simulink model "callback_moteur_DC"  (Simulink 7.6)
settings: Solver=ode15s  StartTime=0.0  StopTime=N  RelTol=1e-3
PostLoadFcn:
  | clc
  | clear all
  | close all
  | delete *.mat
InitFcn:
  | clc, clear all, close all
  | % Durée de simulation et temps de l'échelon
  | N=1;
  | % paramètres du moteur
  | R=3.9; % résistance d'induit
  | L=12e-6; % inductance d'induit
  | K=5e-4; % paramètre électromécanique
  | J=0.02; % inertie
  | Mr=0.02e-3; % frottements
StopFcn:
  | close all
  | load vit_pos_mot_DC.mat
  | plotyy(x(1,:),x(2,:), x(1,:),x(3,:))
  | grid
  | title('Position et Vitesse d''un moteur DC')
  | xlabel('temps')
libraries: fl_lib x10, nesl_utility x4

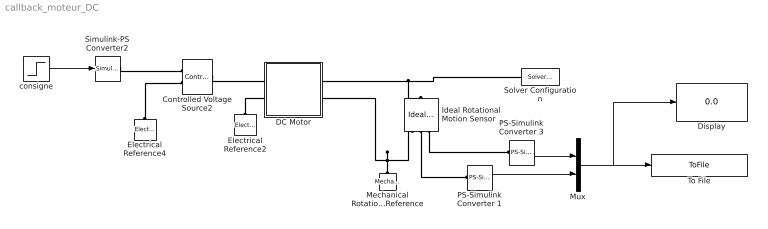
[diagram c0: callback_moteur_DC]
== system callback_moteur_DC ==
  Controlled Voltage Source2 : fl_lib/Electrical/Electrical Sources/Controlled Voltage Source  DialogController=NetworkEngine.DynNeDlgSource  SystemSampleTime=-1  i_Log=off  v_Log=off  LocalVarNames=|current|voltage|power  LocalVarDescs=|Current (A)|Voltage (V)|Power (W)  LocalVarLogging=[0 0 0]
  DC Motor : Subsystem
  Display : Display
  Electrical Reference2 : fl_lib/Electrical/Electrical Elements/Electrical Reference  DialogController=NetworkEngine.DynNeDlgSource  SystemSampleTime=-1  i_Log=off  LocalVarNames=|i  LocalVarDescs=|i  LocalVarLogging=[]
  Electrical Reference4 : fl_lib/Electrical/Electrical Elements/Electrical Reference  DialogController=NetworkEngine.DynNeDlgSource  SystemSampleTime=-1  i_Log=off  LocalVarNames=|i  LocalVarDescs=|i  LocalVarLogging=[]
  Ideal Rotational Motion Sensor : fl_lib/Mechanical/Mechanical Sensors/Ideal Rotational Motion Sensor  DialogController=NetworkEngine.DynNeDlgSource  SystemSampleTime=-1  offset=0 rad  w_Log=off  t_Log=off  phi_Log=off  LocalVarNames=|w|t|phi  LocalVarDescs=|w|t|phi  LocalVarLogging=[]
  Mechanical Rotational Reference : fl_lib/Mechanical/Rotational Elements/Mechanical Rotational Reference  DialogController=NetworkEngine.DynNeDlgSource  SystemSampleTime=-1  t_Log=off  LocalVarNames=|t  LocalVarDescs=|t  LocalVarLogging=[]
  Mux : Mux  Inputs=2
  PS-Simulink Converter 1 : nesl_utility/PS-Simulink Converter  DialogController=NetworkEngine.DynNeUtilDlgSource  SystemSampleTime=-1  PhysicalDomain=network_engine_domain  LeftPortType=input  RightPortType=output  SubClassName=ps_output  Unit=rpm  AffineConversion=off
  PS-Simulink Converter 3 : nesl_utility/PS-Simulink Converter  DialogController=NetworkEngine.DynNeUtilDlgSource  SystemSampleTime=-1  PhysicalDomain=network_engine_domain  LeftPortType=input  RightPortType=output  SubClassName=ps_output  Unit=rad  AffineConversion=off
  Simulink-PS Converter2 : nesl_utility/Simulink-PS Converter  DialogController=NetworkEngine.DynNeUtilDlgSource  SystemSampleTime=-1  PhysicalDomain=network_engine_domain  LeftPortType=input  RightPortType=output  SubClassName=ps_input  Unit=1  AffineConversion=off  InputFilterTimeConstant=.001  UdotUserProvided=0
  Solver Configuration : nesl_utility/Solver Configuration  DialogController=NetworkEngine.DynNeUtilDlgSource  SystemSampleTime=-1  PhysicalDomain=network_engine_domain  LeftPortType=input  RightPortType=generic  SubClassName=solver  Accelerate=off  Profile=off  ResidualTolerance=1e-9  MaxNonlinIter=3  MaxModeIter=2  DoFixedCost=off  UseLocalSampling=off  DoDC=off  LinearAlgebra=Sparse  LocalSolverSampleTime=.001  LocalSolverChoice=NE_BACKWARD_EULER_ADVANCER  UseLocalSolver=off
  To File : ToFile  Filename=vit_pos_mot_DC.mat  MatrixName=x
  consigne : Step  Time=0.2  After=12  SampleTime=0
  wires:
  PS-Simulink Converter 3/1 -> Mux/1
  PS-Simulink Converter 1/1 -> Mux/2
  Mux/1 -> To File/1, Display/1
  consigne/1 -> Simulink-PS Converter2/1
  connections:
  Electrical Reference2/LConn1 -- DC Motor/LConn2
  Mechanical Rotational Reference/LConn1 -- Ideal Rotational Motion Sensor/RConn1 -- DC Motor/RConn2
  DC Motor/RConn1 -- Solver Configuration/RConn1 -- Ideal Rotational Motion Sensor/LConn1
  Ideal Rotational Motion Sensor/RConn2 -- PS-Simulink Converter 1/LConn1
  Ideal Rotational Motion Sensor/RConn3 -- PS-Simulink Converter 3/LConn1
  Electrical Reference4/LConn1 -- Controlled Voltage Source2/RConn2
  Simulink-PS Converter2/RConn1 -- Controlled Voltage Source2/RConn1
  Controlled Voltage Source2/LConn1 -- DC Motor/LConn1

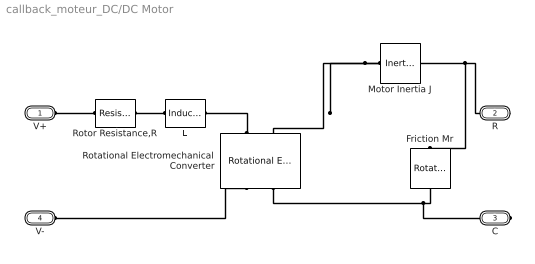
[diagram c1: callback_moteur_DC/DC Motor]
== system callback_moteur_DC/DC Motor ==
  Friction Mr : fl_lib/Mechanical/Rotational Elements/Rotational Friction  DialogController=NetworkEngine.DynNeDlgSource  SystemSampleTime=-1  brkwy_trq=Mr N*m  Col_trq=Mr N*m  visc_coef=0 N*m/(rad/s)  trans_coef=10 s/rad  vel_thr=0.1 rad/s  t_Log=off  w_Log=off  LocalVarNames=|friction_torque|rel_velocity|power  LocalVarDescs=|Friction torque (N*m)|Relative velocity (rad/s)|Power (W)  LocalVarLogging=[0 0 0]
  L : fl_lib/Electrical/Electrical Elements/Inductor  DialogController=NetworkEngine.DynNeDlgSource  SystemSampleTime=-1  l=L H  i0=0 A  r=0 Ohm  g=1e-09 1/Ohm  i_Log=off  v_Log=off  i_L_Log=off  LocalVarNames=|current|voltage|power  LocalVarDescs=|Inductor current (A) |Voltage across inductor (V)|Power (W)  LocalVarLogging=[0 0 0]
  Motor Inertia J : fl_lib/Mechanical/Rotational Elements/Inertia  DialogController=NetworkEngine.DynNeDlgSource  SystemSampleTime=-1  inertia=J g*cm^2  initial_velocity=0 rad/s  t_Log=off  LocalVarNames=|torque|velocity  LocalVarDescs=|Inertia torque (N*m)|Inertia absolute velocity (rad/s)  LocalVarLogging=[0 0]
  Rotational Electromechanical Converter : fl_lib/Electrical/Electrical Elements/Rotational Electromechanical Converter  DialogController=NetworkEngine.DynNeDlgSource  SystemSampleTime=-1  K=K V/(rad/s)  i_Log=off  v_Log=off  t_Log=off  w_Log=off  LocalVarNames=|current|voltage|power|torque|speed  LocalVarDescs=|Current (A)|Voltage (V)|Power (W)|Torque (Nm)|Angular speed (rad/s)  LocalVarLogging=[0 0 0 0 0]
  Rotor Resistance,R : fl_lib/Electrical/Electrical Elements/Resistor  Tag=Factory Generic  DialogController=NetworkEngine.DynNeDlgSource  SystemSampleTime=-1  R=R Ohm  i_Log=off  v_Log=off  LocalVarNames=|current|voltage|power  LocalVarDescs=|Resistor current (A)|Voltage across resistor (V)|Power (W)  LocalVarLogging=[0 0 0]
  V+ : PMIOPort  Port=1  Side=Left
  R : PMIOPort  Port=2  Side=Right
  C : PMIOPort  Port=3  Side=Right
  V- : PMIOPort  Port=4  Side=Left
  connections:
  Rotational Electromechanical Converter/LConn1 -- L/RConn1
  V-/RConn1 -- Rotational Electromechanical Converter/RConn1
  Rotor Resistance,R/LConn1 -- V+/RConn1
  L/LConn1 -- Rotor Resistance,R/RConn1
  Motor Inertia J/LConn1 -- Rotational Electromechanical Converter/LConn2 -- R/RConn1 -- Friction Mr/LConn1
  Rotational Electromechanical Converter/RConn2 -- C/RConn1 -- Friction Mr/RConn1
